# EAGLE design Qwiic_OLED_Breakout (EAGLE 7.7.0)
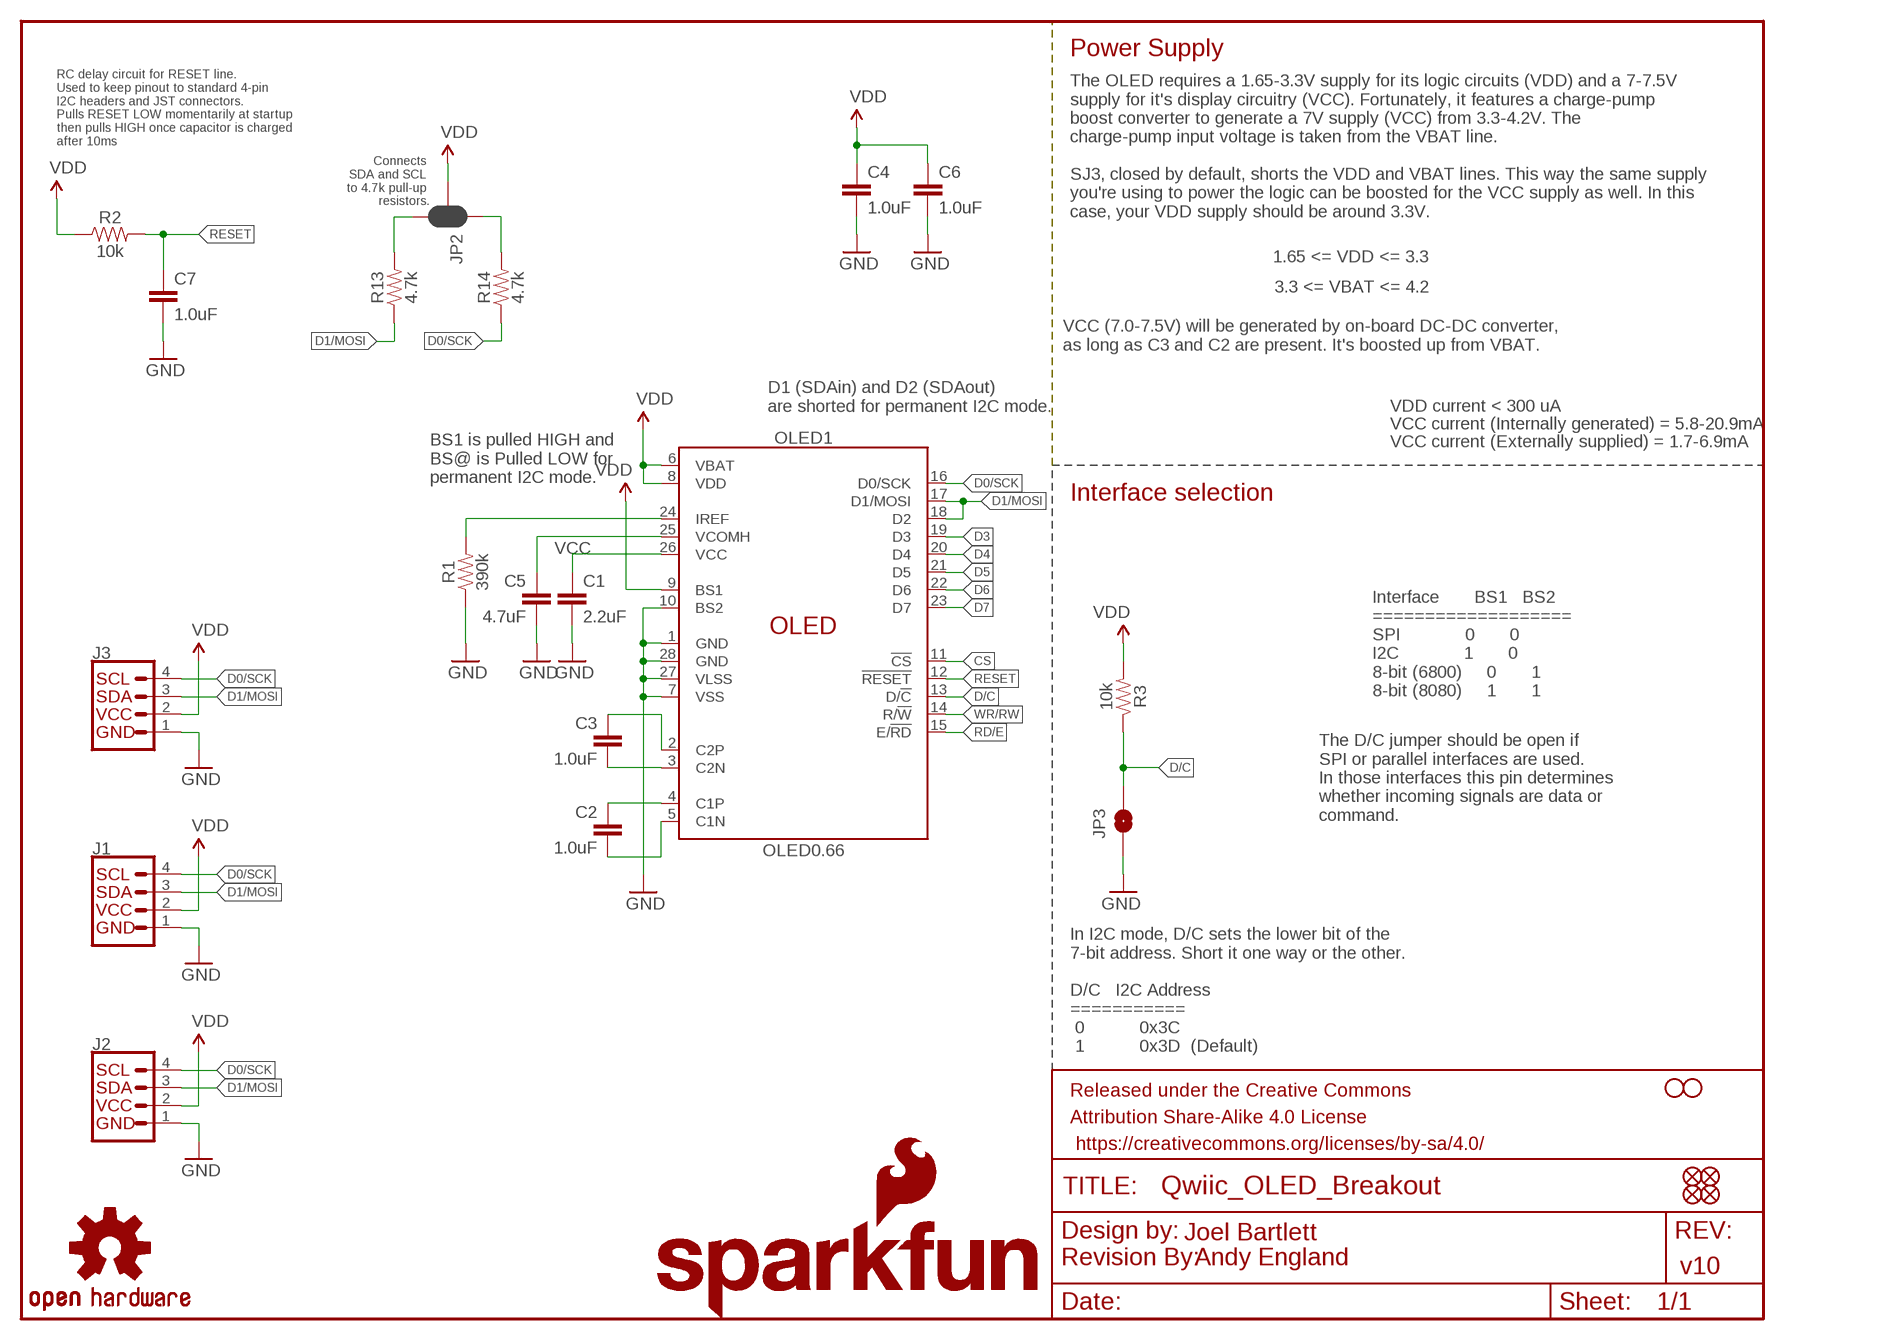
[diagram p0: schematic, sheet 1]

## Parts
C1  2.2uF  2.2UF-0805-25V-(+80/-20%)  [0805]
C2  1.0uF  1.0UF-0805-25V-10%  [0805]
C3  1.0uF  1.0UF-0805-25V-10%  [0805]
C4  1.0uF  1.0UF-0603-16V-10%  [0603]
C5  4.7uF  4.7UF-1206-16V-(+80/-20%)  [1206]
C6  1.0uF  1.0UF-0603-16V-10%  [0603]
C7  1.0uF  1.0UF-0603-16V-10%  [0603]
FID1  FIDUCIAL1X2  [FIDUCIAL-1X2]
FID2  FIDUCIAL1X2  [FIDUCIAL-1X2]
FID3  FIDUCIAL1X2  [FIDUCIAL-1X2]
FID4  FIDUCIAL1X2  [FIDUCIAL-1X2]
FRAME1  FRAME-LETTER  [CREATIVE_COMMONS]
H1  STAND-OFF  [STAND-OFF]
H2  STAND-OFF  [STAND-OFF]
J1  QWIIC_CONNECTORJS-1MM  [1X04_1MM_RA]
J2  QWIIC_CONNECTORJS-1MM  [1X04_1MM_RA]
J3  I2C_STANDARD_NO_SILK  [1X04_NO_SILK]
JP2  JUMPER-SMT_3_2-NC_PASTE_SILK  [SMT-JUMPER_3_2-NC_PASTE_SILK]
JP3  JUMPER-SMT_2_NO_SILK  [SMT-JUMPER_2_NO_SILK]
LOGO1  REVISION  [REVISION]
LOGO2  SFE_LOGO_FLAME.1_INCH  [SFE_LOGO_FLAME_.1]
LOGO3  OSHW-LOGOS  [OSHW-LOGO-S]
LOGO4  SFE_LOGO_NAME.1_INCH  [SFE_LOGO_NAME_.1]
OLED1  OLED0.66  [OLED-0.66-64X48]
R1  390k  390KOHM-0603-1/10W-1%  [0603]
R2  10k  10KOHM-0603-1/10W-1%  [0603]
R3  10k  10KOHM-0603-1/10W-1%  [0603]
R13  4.7k  4.7KOHM-0603-1/10W-1%  [0603]
R14  4.7k  4.7KOHM-0603-1/10W-1%  [0603]

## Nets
C1P: C2.1 OLED1.4(C1P)
C2N: C3.2 OLED1.3(C2N)
CS: OLED1.11(!CS!)
D0/SCK: J1.4 J2.4 J3.4(SCL) OLED1.16(D0/SCK) R14.1
D1/MOSI: J1.3 J2.3 J3.3(SDA) OLED1.17(D1/MOSI) OLED1.18(D2) R13.1
D3: OLED1.19(D3)
D4: OLED1.20(D4)
D5: OLED1.21(D5)
D6: OLED1.22(D6)
D7: OLED1.23(D7)
D/C: JP3.2 OLED1.13(D/!C!) R3.1
GND: C1.2 C4.2 C5.2 C6.2 C7.2 J1.1 J2.1 J3.1(GND) JP3.1 OLED1.1(GND) OLED1.7(VSS) OLED1.10(BS2) OLED1.27(VLSS) OLED1.28(GND) R1.1
IREF: OLED1.24(IREF) R1.2
N$1: C3.1 OLED1.2(C2P)
N$2: C2.2 OLED1.5(C1N)
N$4: JP2.3 R13.2
N$5: JP2.1 R14.2
RD/E: OLED1.15(E/!RD!)
RESET: C7.1 OLED1.12(!RESET!) R2.2
VCC: C1.1 OLED1.26(VCC)
VCOMH: C5.1 OLED1.25(VCOMH)
VDD: C4.1 C6.1 J1.2 J2.2 J3.2(VCC) JP2.2 OLED1.6(VBAT) OLED1.8(VDD) OLED1.9(BS1) R2.1 R3.2
WR/RW: OLED1.14(R/!W!)

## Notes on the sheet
- Power Supply
- The OLED requires a 1.65-3.3V supply for its logic circuits (VDD) and a 7-7.5V
  supply for it's display circuitry (VCC). Fortunately, it features a charge-pump 
  boost converter to generate a 7V supply (VCC) from 3.3-4.2V. The 
  charge-pump input voltage is taken from the VBAT line.
  
  SJ3, closed by default, shorts the VDD and VBAT lines. This way the same supply 
  you're using to power the logic can be boosted for the VCC supply as well. In this 
  case, your VDD supply should be around 3.3V.
- RC delay circuit for RESET line. 
  Used to keep pinout to standard 4-pin
  I2C headers and JST connectors. 
  Pulls RESET LOW momentarily at startup
  then pulls HIGH once capacitor is charged
  after 10ms
- Connects 
  SDA and SCL 
  to 4.7k pull-up 
  resistors.
- 1.65 <= VDD <= 3.3
- 3.3 <= VBAT <= 4.2
- VCC (7.0-7.5V) will be generated by on-board DC-DC converter, 
  as long as C3 and C2 are present. It's boosted up from VBAT.
- D1 (SDAin) and D2 (SDAout)
  are shorted for permanent I2C mode.
- VDD current < 300 uA
- VCC current (Internally generated) = 5.8-20.9mA
- VCC current (Externally supplied) = 1.7-6.9mA
- BS1 is pulled HIGH and 
  BS@ is Pulled LOW for 
  permanent I2C mode.
- Interface selection
- Interface       BS1   BS2
  ===================
  SPI             0       0
  I2C             1       0
  8-bit (6800)     0       1
  8-bit (8080)     1       1
- The D/C jumper should be open if
  SPI or parallel interfaces are used.
  In those interfaces this pin determines
  whether incoming signals are data or
  command.
- In I2C mode, D/C sets the lower bit of the 
  7-bit address. Short it one way or the other.
  
  D/C   I2C Address
  ===========
   0           0x3C
   1           0x3D  (Default)
- Joel Bartlett
- Andy England
- v10

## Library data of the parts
C1 = SparkFun-Capacitors:2.2UF: 2.2µF ceramic capacitors; PROD_ID: CAP-11624
C2 C3 = SparkFun-Capacitors:1.0UF: 1µF ceramic capacitors; PROD_ID: CAP-08064
C4 C6 C7 = SparkFun-Capacitors:1.0UF: 1µF ceramic capacitors; PROD_ID: CAP-00868
C5 = SparkFun-Capacitors:4.7UF: 4.7µF ceramic capacitors; PROD_ID: CAP-10300
FID1-FID4 = SparkFun-Aesthetics:FIDUCIAL: Fiducial Alignment Points
FRAME1 = SparkFun-Aesthetics:FRAME-LETTER: Schematic Frame
H1 H2 = SparkFun-Hardware:STAND-OFF: Stand Off
J1 J2 = SparkFun-Connectors:QWIIC_CONNECTOR: SparkFun I2C Standard Qwiic Connector An SMD 1mm pitch JST connector makes it easy and quick (get it? Qwiic?) to connect I2C devices to each other. The Qwiic system enables fast and solderless connection between popular platforms and various sensors and actuators. We carry 200mm, 100mm, 50mm, and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; PROD_ID: CONN-13694
J3 = SparkX:I2C_STANDARD: SparkFun I2C Standard Pinout Header SparkFun has standardized on a pinout for all I2C based sensor breakouts. This pinout allows I2C boards to be plugged directly into the headers on Arduino Uno compatible boards, and to be daisy chained easily. Example SparkFun Products: SparkFun Atmospheric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
JP2 = SparkFun-Jumpers:JUMPER-SMT_3_2-NC_PASTE: Normally closed solder jumper (2 of 2 connections) This jumper has an aperture in the stencil to allow solder paste to bridge both connections. Both connections are normally closed (NC). Wick off the solder to open the connection(s). Reapply solder to reclose the connection(s).
JP3 = SparkFun-Jumpers:JUMPER-SMT_2_NO: Normally open jumper
LOGO1 = SparkFun-Aesthetics:REVISION: "Revision By" Text
LOGO2 = SparkFun-Aesthetics:SFE_LOGO_FLAME: SparkFun Flame Logo
LOGO3 = SparkFun-Aesthetics:OSHW-LOGO: Open Source Hardware Logo This logo indicates the piece of hardware it is found on incorporates a OSHW license and/or adheres to the definition of open source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
LOGO4 = SparkFun-Aesthetics:SFE_LOGO_NAME: SparkFun Font Logo
OLED1 = SparkFun-Displays:OLED0.66: Micro OLED TODO: Add description SparkFun Products: Micro OLED Breakout; PROD_ID: LCD-12019
R1 = SparkFun-Resistors:390KOHM: 390kΩ resistor; PROD_ID: RES-12024
R2 R3 = SparkFun-Resistors:10KOHM: 10kΩ resistor; PROD_ID: RES-00824
R13 R14 = SparkFun-Resistors:4.7KOHM: 4.7kΩ resistor; PROD_ID: RES-07857

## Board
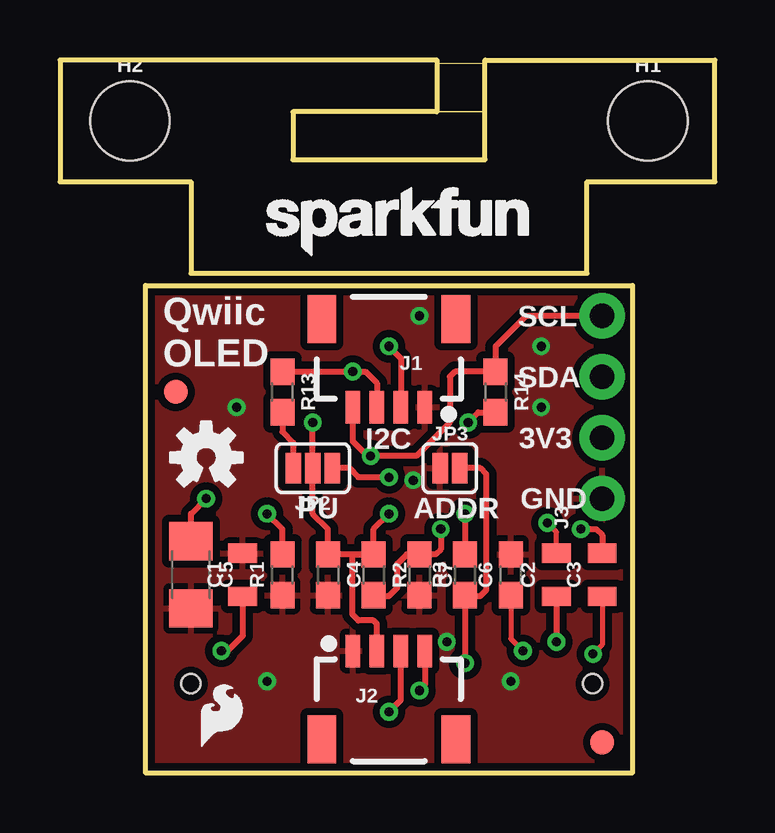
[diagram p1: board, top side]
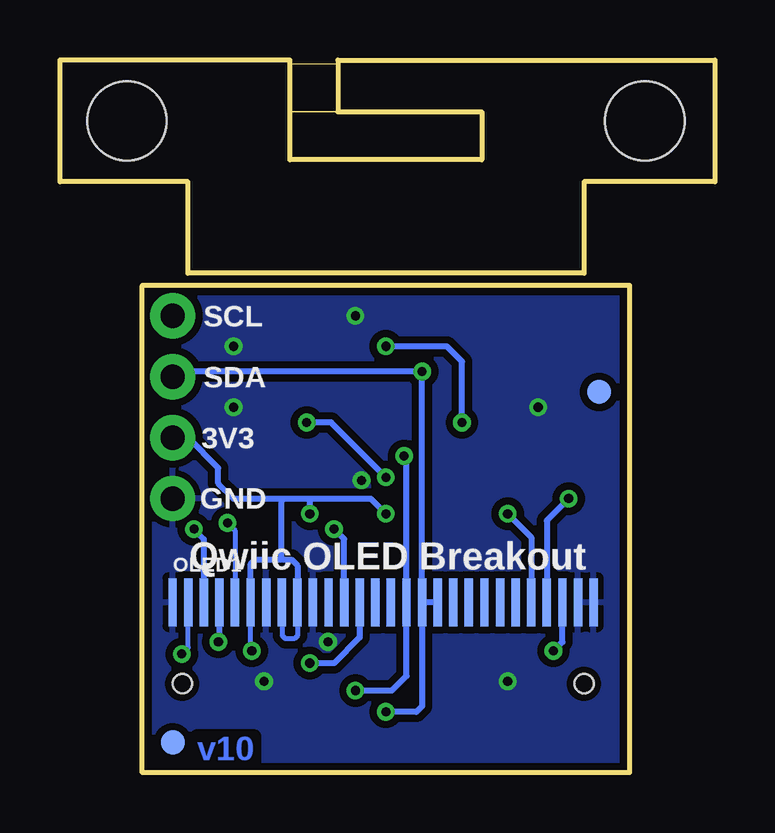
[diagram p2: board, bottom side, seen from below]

Size 27.3 x 29.72 mm. Coordinates in mm from the lower left corner, seen from the top.
Outline: 17.72,25.56 9.72,25.56 9.72,27.56 15.72,27.56 15.72,29.72 0,29.72 0,24.64 5.46,24.64 5.46,20.83 21.97,20.83 21.97,24.64 27.3,24.64 27.3,29.72 17.72,29.72 17.72,25.56
Outline: 23.88,0 23.88,20.32 3.56,20.32 3.56,0 23.88,0
Copper layers (1*16): Top 0.035mm / dielectric 1.5mm / Bottom 0.035mm
Design rules "SparkFun-2-layer-TIGHT": minimum track width 7mil, minimum drill 15mil, track to track 7mil, track to pad 7mil, pad to pad 7mil, via to via 7mil, smd to smd 7mil, copper to edge 7mil, drill to drill 7mil, minimum pad ring 7mil, minimum via ring 7mil, stop-mask expansion 4mil, vias tented up to drill 25mil, thermal gap 10mil
Milling: area 9.7,25.6 to 17.7,27.6; area 15.7,27.6 to 17.7,29.6

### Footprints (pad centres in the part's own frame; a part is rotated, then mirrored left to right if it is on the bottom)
0805 = smd 0.8 x 1.2: 1 -0.9,0; 2 0.9,0
0603 = smd 1.1 x 1: 1 -0.85,0; 2 0.85,0
1206 = smd 1.6 x 1.8: 1 -1.4,0; 2 1.4,0
FIDUCIAL-1X2 = smd 1 x 1: 1 0,0
STAND-OFF = hole 3.302: 0,0
1X04_1MM_RA = smd 0.6 x 1.35: 1 -1.5,0; 2 -0.5,0; 3 0.5,0; 4 1.5,0 | smd 1.2 x 2: NC1 2.8,-3.675; NC2 -2.8,-3.675
1X04_NO_SILK = drill 1.016 pad 1.88: 1 0,0; 2 2.54,0; 3 5.08,0; 4 7.62,0
SMT-JUMPER_3_2-NC_PASTE_SILK = smd 0.635 x 1.27: 1 -0.813,0; 2 0,0; 3 0.813,0
SMT-JUMPER_2_NO_SILK = smd 0.635 x 1.27: 1 -0.406,0; 2 0.406,0
OLED-0.66-64X48 = smd 0.35 x 2: 1 0,0; 2 0.65,0; 3 1.3,0; 4 1.95,0; 5 2.6,0; 6 3.25,0; 7 3.9,0; 8 4.55,0; 9 5.2,0; 10 5.85,0; 11 6.5,0; 12 7.15,0; 13 7.8,0; 14 8.45,0; 15 9.1,0; 16 9.75,0; 17 10.4,0; 18 11.05,0; 19 11.7,0; 20 12.35,0; 21 13,0; 22 13.65,0; 23 14.3,0; 24 14.95,0; 25 15.6,0; 26 16.25,0; 27 16.9,0; 28 17.55,0 | hole 0.8: 17.15,-3.4; 0.4,-3.4

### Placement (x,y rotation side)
C1  7.62,8.26 90 top
C2  20.7,8.26 90 top
C3  22.61,8.26 90 top
C4  11.18,8.26 270 top
C5  5.46,8.26 270 top
C6  18.8,8.26 90 top
C7  14.99,8.26 270 top
FID1  22.61,1.27 0 top
FID2  4.83,15.88 0 top
FID3  4.83,15.88 0 bottom
FID4  22.61,1.27 0 bottom
FRAME1  not placed on the board
H1  24.51,27.18 0 top
H2  2.92,27.18 0 top
J1  13.72,15.24 180 top
J2  13.72,5.08 0 top
J3  22.61,11.43 90 top
JP2  10.54,12.7 180 top
JP3  16.26,12.7 0 top
LOGO1  not placed on the board
LOGO2  5.59,0.76 0 top
LOGO3  6.1,13.14 0 top
LOGO4  8.13,21.08 0 top
OLED1  22.61,7.11 0 bottom
R1  9.27,8.26 90 top
R2  13.08,8.26 270 top
R3  16.89,8.26 90 top
R13  9.27,15.88 270 top
R14  18.16,15.88 270 top

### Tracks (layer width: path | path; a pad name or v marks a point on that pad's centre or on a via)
C1P  (via drill 0.38)
  Top 0.254: C2.1 v20.7,5.46
  Bottom 0.254: v20.7,5.46 20.66,5.51 OLED1.4
C2N  (via drill 0.38)
  Top 0.254: 22.61,9.53 C3.2 22.61,9.91 22.35,10.16 v21.72,10.16
  Bottom 0.254: OLED1.3 21.31,9.75 v21.72,10.16
D0/SCK  (via drill 0.38)
  Top 0.254: J2.4 15.22,3.66 v14.99,3.43 | J3.4 19.43,19.05 18.16,17.78 R14.1 16.47,16.73 16.26,16.51 16.26,14.61 14.86,13.21 v12.95,13.21 12.83,13.21 12.22,13.82 J1.4
  Bottom 0.254: v14.99,3.43 13.46,3.43 12.86,4.04 OLED1.16 12.86,13.11 v12.95,13.21
D1/MOSI  (via drill 0.38)
  Top 0.254: v13.72,2.54 14.22,3.04 J2.3 | R13.1 v12.21,16.73 12.74,16.73 13.22,16.25 J1.3
  Bottom 0.254: OLED1.18 OLED1.17 | OLED1.17 12.21,2.78 12.45,2.54 v13.72,2.54 | OLED1.17 v12.21,16.73 22.39,16.73 J3.3
D/C  (via drill 0.38)
  Top 0.254: R3.1 16.93,7.37 | 16.93,7.37 17.53,7.37 17.78,7.62 17.78,12.45 17.53,12.7 JP3.2 | 16.93,7.37 16.89,7.33 v16.89,4.57
  Bottom 0.254: OLED1.13 14.81,5.64 15.88,4.57 v16.89,4.57
GND  (via drill 0.38)
  other vias: 8.64,3.81 14.73,12.19 20.07,15.24 14.99,19.05 20.07,17.78 18.8,3.81 7.37,15.24 16.13,5.46
  pour Bottom (isolate 0.305): 23.88,0 23.88,20.32 3.56,20.32 3.56,0
  pour Top (isolate 0.305): 23.88,0 23.88,20.32 3.56,20.32 3.56,0
IREF  (via drill 0.38)
  Top 0.254: R1.2 9.27,10.16 v8.64,10.79
  Bottom 0.254: v8.64,10.79 7.66,9.81 OLED1.24
N$1  (via drill 0.38)
  Top 0.203: C3.1 22.61,5.33 v22.23,4.95
  Bottom 0.203: v22.23,4.95 21.96,5.22 OLED1.2
N$2  (via drill 0.38)
  Top 0.203: C2.2 20.7,10.03 v20.32,10.41
  Bottom 0.203: v20.32,10.41 20.01,10.1 OLED1.5
N$4
  Top 0.254: R13.2 9.27,14.22 9.73,13.77 JP2.3
N$5  (via drill 0.38)
  Top 0.254: 17.95,15.03 R14.2 17.44,15.03 v17.02,14.61 | v13.72,12.32 12.45,12.32 12.07,12.7 JP2.1
  Bottom 0.254: v13.72,12.32 16,14.61 v17.02,14.61
RESET  (via drill 0.38)
  Top 0.254: R2.2 13.12,7.37 13.72,7.37 14.07,7.72 14.07,8.71 14.46,9.11 C7.1 15.66,9.11 15.88,9.32 v15.88,10.16
  Bottom 0.254: OLED1.12 15.46,9.74 v15.88,10.16
VCC  (via drill 0.38)
  Top 0.254: C1.1 7.62,5.71 6.98,5.08 v6.73,5.08
  Bottom 0.254: v6.73,5.08 6.36,5.46 OLED1.26
VCOMH  (via drill 0.38)
  Top 0.254: C5.1 5.46,10.79 v6.1,11.43
  Bottom 0.254: v6.1,11.43 7.01,10.52 OLED1.25
VDD  (via drill 0.38)
  Top 0.203: C6.1 18.8,5.59 v19.3,5.08
  Top 0.254: J2.2 13.22,6.21 13.08,6.35 12.45,6.35 12.19,6.6 12.19,9.11 R2.1 | R2.1 C4.1 11.18,10.16 10.54,10.79 JP2.2 v10.54,14.61 | v16.89,10.79 R3.2 | v13.72,17.78 14.22,17.28 J1.2 | R2.1 13.08,10.16 v13.72,10.79
  Bottom 0.203: OLED1.9 17.41,5.71 17.53,5.59 17.91,5.59 18.03,5.71 18.03,7.09 OLED1.8 | v19.3,5.08 19.36,5.13 OLED1.6
  Bottom 0.254: 18.06,8.89 18.06,11.32 18.16,11.43 | v10.54,14.61 10.54,17.14 11.18,17.78 v13.72,17.78 | 16.89,11.43 v16.89,10.79 | 18.16,11.43 20.07,11.43 20.7,12.06 20.7,12.7 21.97,13.97 J3.2 | 18.16,11.43 16.89,11.43 | 16.89,11.43 14.35,11.43 v13.72,10.79 | 18.06,8.89 17.65,8.89 17.41,8.64 OLED1.9 | OLED1.6 19.36,8.71 19.18,8.89 18.06,8.89

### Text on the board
Bottom: v10
tPlace: SCL | Qwiic / OLED | SDA | 3V3 | I2C | PU | ADDR | GND
bPlace: SCL | SDA | 3V3 | GND | Qwiic OLED Breakout
tDocu: Joel Bartlett | Andy England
